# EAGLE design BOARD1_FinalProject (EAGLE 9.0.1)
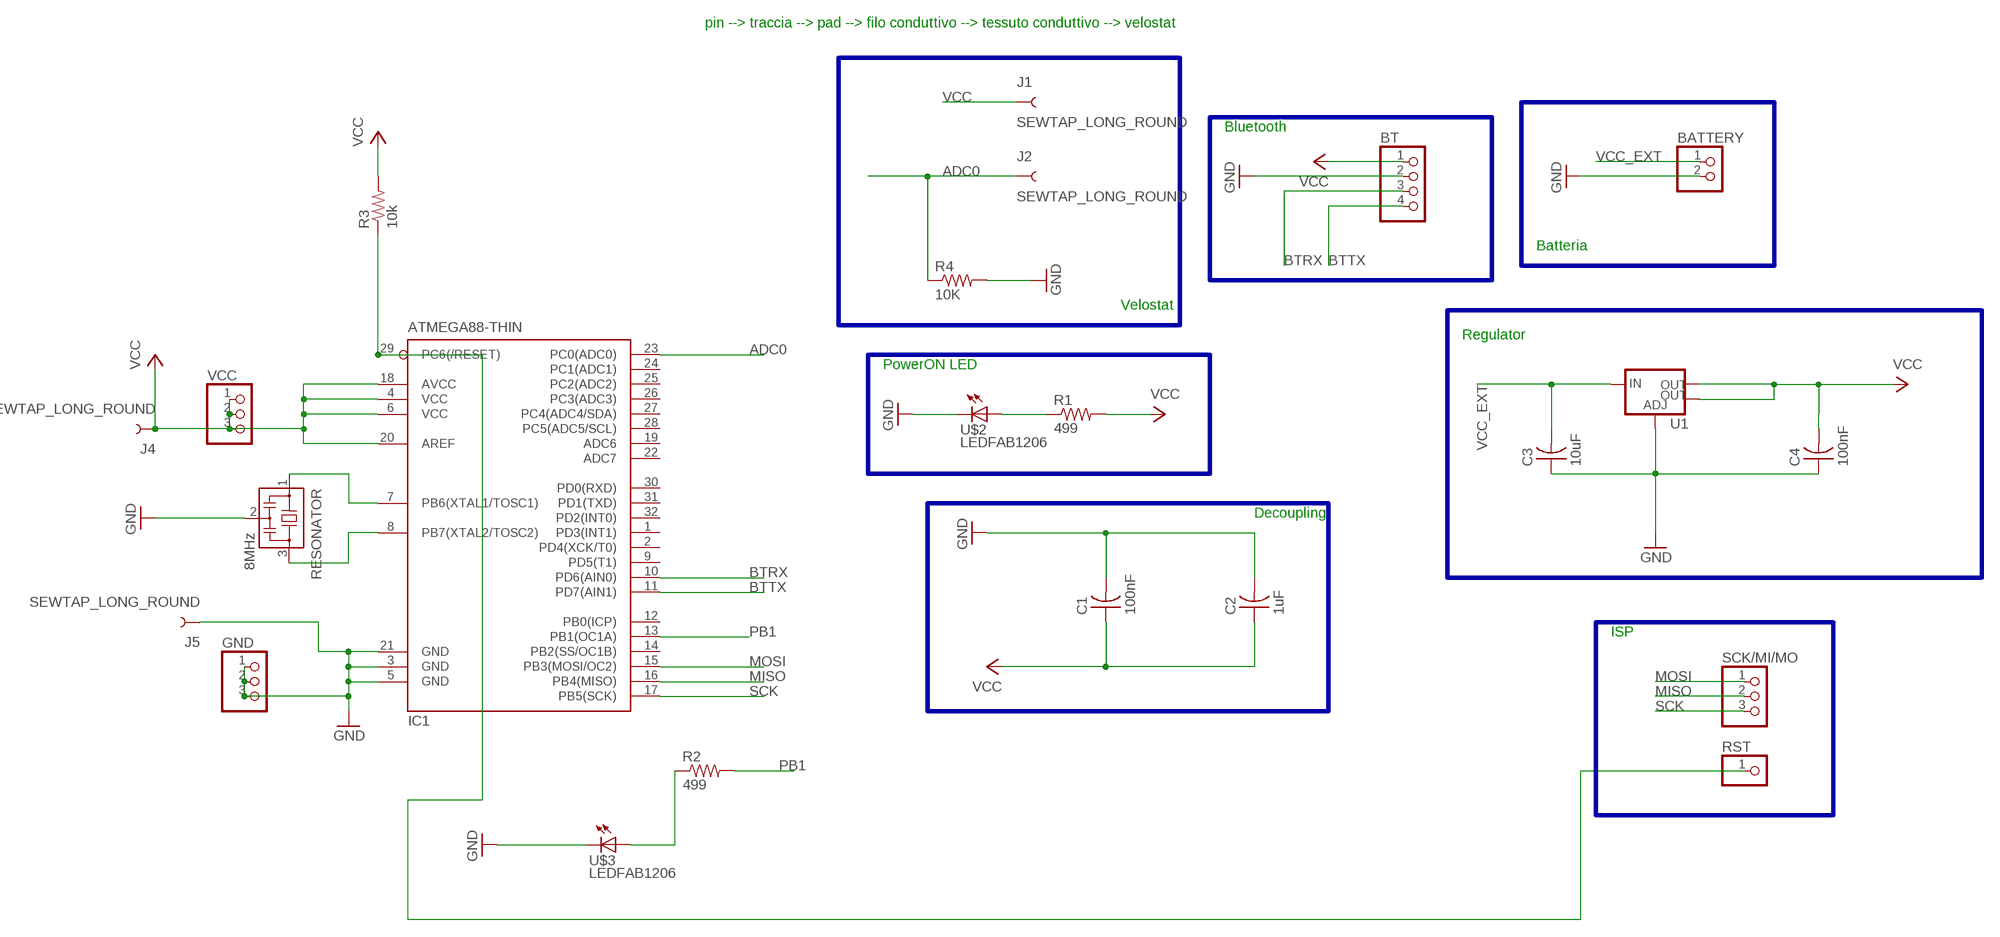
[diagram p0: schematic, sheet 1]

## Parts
BATTERY  PINHD-1X2  [1X02]
BT  PINHD-1X4  [1X04]
C1  100nF  CAP-US1206FAB  [C1206FAB]
C2  1uF  CAP-US1206FAB  [C1206FAB]
C3  10uF  CAP-US1206FAB  [C1206FAB]
C4  100nF  CAP-US1206FAB  [C1206FAB]
GND  PINHD-1X3  [1X03]
IC1  ATMEGA88-THIN  [TQFP32-08THIN]
J1  SEWTAP_LONG_ROUND  [PETAL-LONG-2]
J2  SEWTAP_LONG_ROUND  [PETAL-LONG-2]
J4  SEWTAP_LONG_ROUND  [PETAL-LONG-2]
J5  SEWTAP_LONG_ROUND  [PETAL-LONG-2]
R1  499  RES-US1206FAB  [R1206FAB]
R2  499  RES-US1206FAB  [R1206FAB]
R3  10k  RES-US1206FAB  [R1206FAB]
R4  10K  RES-US1206FAB  [R1206FAB]
RESONATOR  8MHz  RESONATOR  [EFOBM]
RST  PINHD-1X1  [1X01]
SCK/MI/MO  PINHD-1X3  [1X03]
U1  V_REG_LM1117SOT223  [SOT223]
U$2  LEDFAB1206  [LED1206FAB]
U$3  LEDFAB1206  [LED1206FAB]
VCC  PINHD-1X3  [1X03]

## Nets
ADC0: IC1.23(PC0(ADC0)) J2.1 R4.1
BTRX: BT.3 IC1.10(PD6(AIN0))
BTTX: BT.4 IC1.11(PD7(AIN1))
GND: BATTERY.2 BT.2 C1.2 C2.2 C3.1 C4.1 GND.1 GND.2 GND.3 IC1.3(GND) IC1.5(GND) IC1.21(GND) J5.1 R4.2 RESONATOR.2 U1.1(ADJ) U$2.2(C) U$3.2(C)
MISO: IC1.16(PB4(MISO)) SCK/MI/MO.2
MOSI: IC1.15(PB3(MOSI/OC2)) SCK/MI/MO.1
N$2: IC1.29(PC6(/RESET)) R3.1 RST.1
N$4: R2.1 U$3.1(A)
N$5: R1.1 U$2.1(A)
N$7: IC1.7(PB6(XTAL1/TOSC1)) RESONATOR.1
N$8: IC1.8(PB7(XTAL2/TOSC2)) RESONATOR.3
PB1: IC1.13(PB1(OC1A)) R2.2
SCK: IC1.17(PB5(SCK)) SCK/MI/MO.3
VCC: BT.1 C1.1 C2.1 C4.2 IC1.4(VCC) IC1.6(VCC) IC1.18(AVCC) IC1.20(AREF) J1.1 J4.1 R1.2 R3.2 U1.2(OUT) U1.4(OUT) VCC.1 VCC.2 VCC.3
VCC_EXT: BATTERY.1 C3.2 U1.3(IN)
Unconnected: IC1.1(PD3(INT1)) IC1.2(PD4(XCK/T0)) IC1.9(PD5(T1)) IC1.12(PB0(ICP)) IC1.14(PB2(SS/OC1B)) IC1.19(ADC6) IC1.22(ADC7) IC1.24(PC1(ADC1)) IC1.25(PC2(ADC2)) IC1.26(PC3(ADC3)) IC1.27(PC4(ADC4/SDA)) IC1.28(PC5(ADC5/SCL)) IC1.30(PD0(RXD)) IC1.31(PD1(TXD)) IC1.32(PD2(INT0))

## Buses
B$1
B$2
B$4
B$5
B$6
B$8
B$3

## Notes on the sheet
- pin --> traccia --> pad --> filo conduttivo --> tessuto conduttivo --> velostat
- Bluetooth
- Batteria
- Velostat
- Regulator
- PowerON LED
- Decoupling
- ISP

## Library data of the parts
BATTERY = pinhead:PINHD-1X2: PIN HEADER
BT = pinhead:PINHD-1X4: PIN HEADER
C1-C4 = fab:CAP-US
GND SCK/MI/MO VCC = pinhead:PINHD-1X3: PIN HEADER
IC1 = fab:ATMEGA88-THIN
J1 J2 J4 J5 = LilyPad-Wearables:SEWTAP: SparkFun LilyPad Sew Taps
R1-R4 = fab:RES-US: Resistor (US Symbol)
RESONATOR = fab:RESONATOR
RST = pinhead:PINHD-1X1: PIN HEADER
U1 = fab:V_REG_LM1117: Voltage Regulator LM1117 Standard adjustable voltage regulator but in SMD form. Spark Fun Electronics SKU : COM-00595; PROD_ID: VREG-08170
U$2 U$3 = fab:LED: LED

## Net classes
0 default: clearance 0.205 mm

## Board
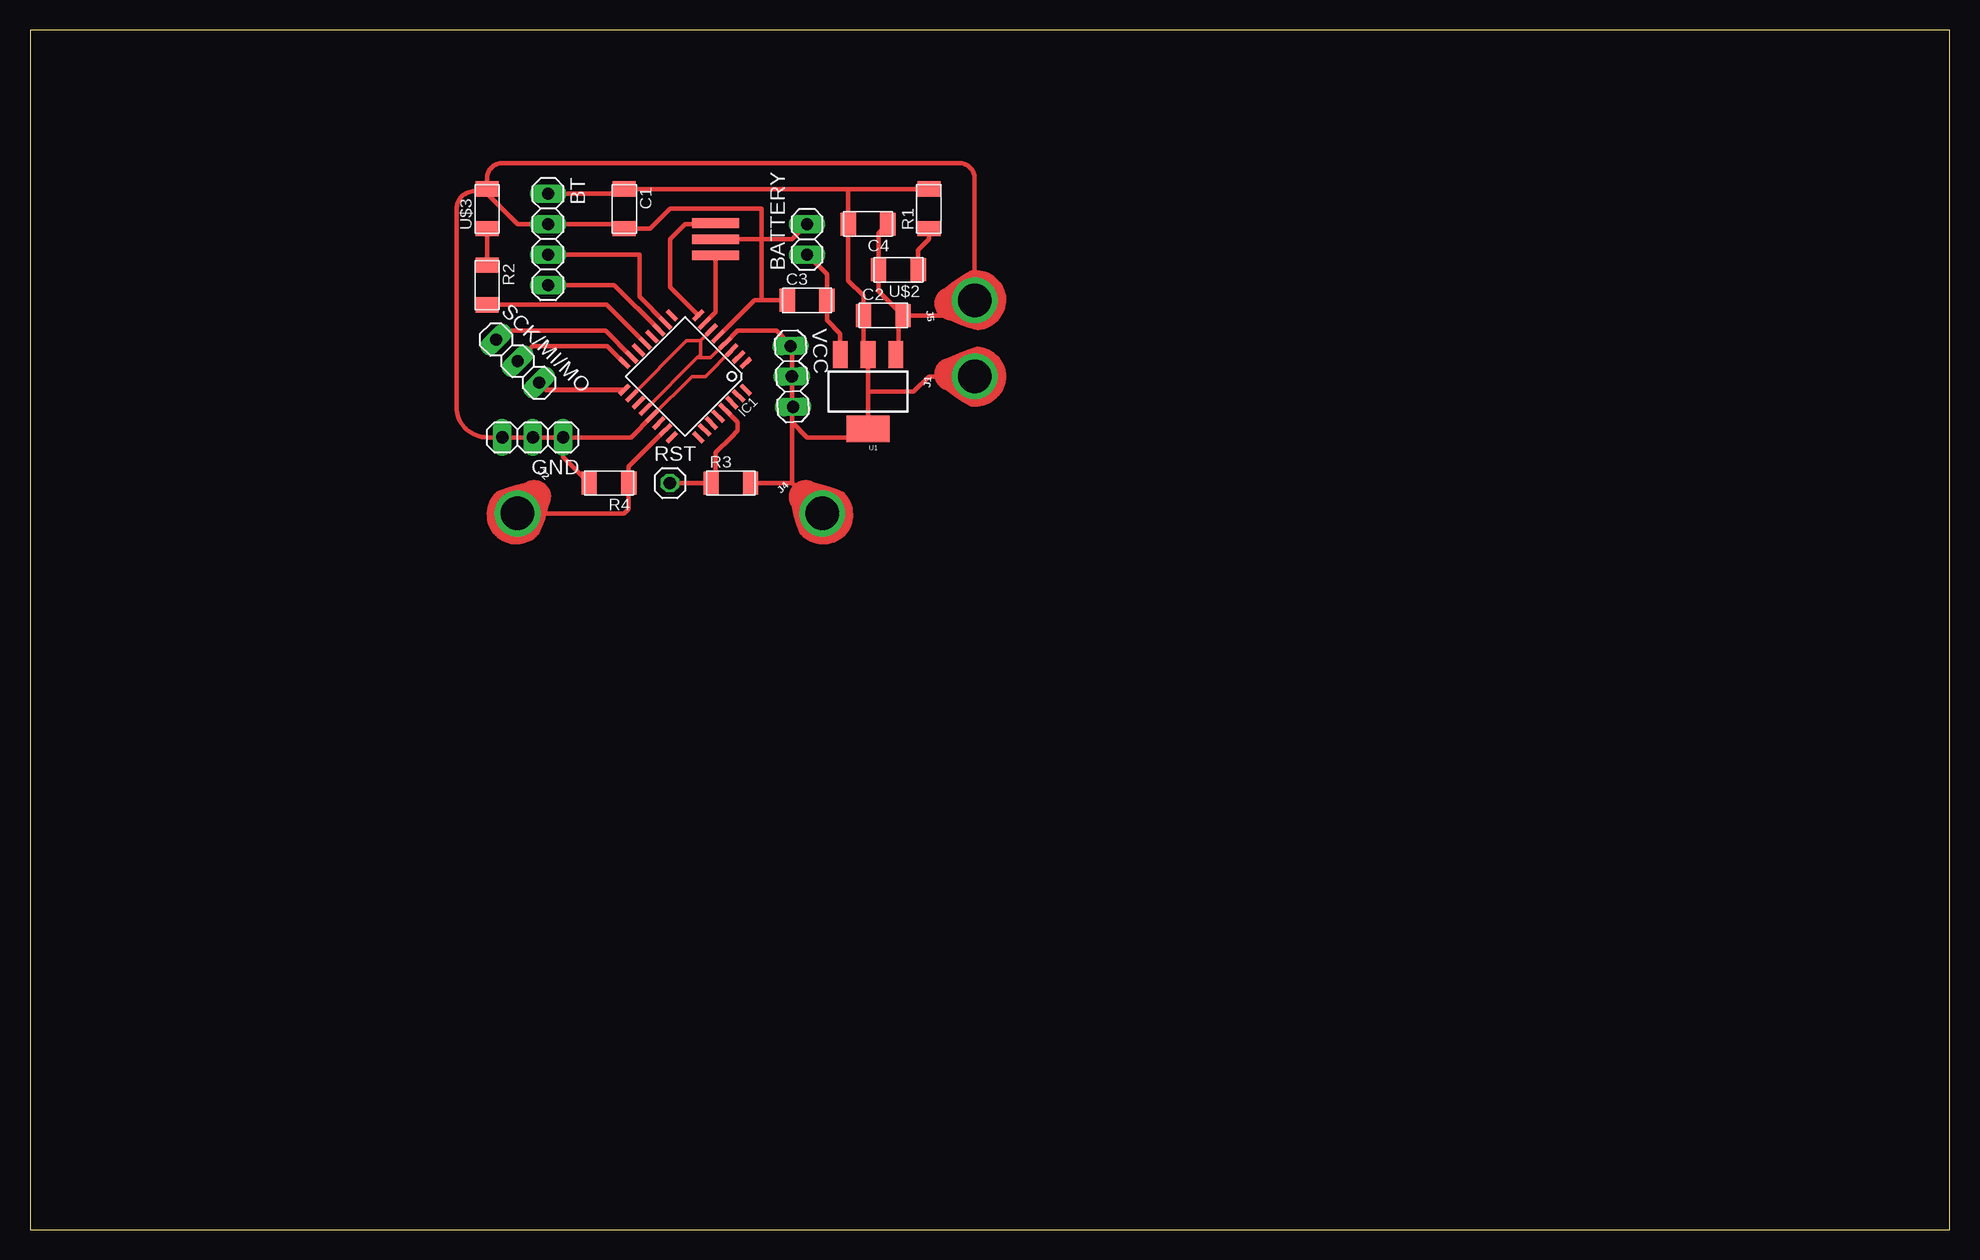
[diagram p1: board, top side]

Size 160 x 100 mm. Coordinates in mm from the lower left corner, seen from the top.
Outline: 0,0 160,0 160,100 0,100 0,0
Copper layers (1*16): Top 0.035mm / dielectric 1.5mm / Bottom 0.035mm
Design rules "default": minimum track width 6mil, minimum drill 0.35mm, track to track 6mil, track to pad 6mil, pad to pad 6mil, via to via 6mil, smd to smd 6mil, copper to edge 40mil, drill to drill 6mil, minimum pad ring 10mil, minimum via ring 8mil, stop-mask expansion 4mil, vias tented up to drill 0mil, thermal gap 10mil

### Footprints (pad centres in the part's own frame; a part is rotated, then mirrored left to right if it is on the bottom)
1X02 = drill 1.016 long: 1 -1.27,0; 2 1.27,0
1X04 = drill 1.016 long: 1 -3.81,0; 2 -1.27,0; 3 1.27,0; 4 3.81,0
C1206FAB = smd 1.27 x 1.905: 1 -1.651,0; 2 1.651,0
1X03 = drill 1.016 long: 1 -2.54,0; 2 0,0; 3 2.54,0
TQFP32-08THIN = smd 1.118 x 0.356: 1 -4.369,2.8; 8 -4.369,-2.8; 17 4.369,-2.8; 24 4.369,2.8 | smd 1.27 x 0.356: 2 -4.293,2; 3 -4.293,1.2; 4 -4.293,0.4; 5 -4.293,-0.4; 6 -4.293,-1.2; 7 -4.293,-2; 18 4.293,-2; 19 4.293,-1.2; 20 4.293,-0.4; 21 4.293,0.4; 22 4.293,1.2; 23 4.293,2 | smd 0.356 x 1.118: 9 -2.8,-4.369; 16 2.8,-4.369; 25 2.8,4.369; 32 -2.8,4.369 | smd 0.356 x 1.27: 10 -2,-4.293; 14 1.2,-4.293; 15 2,-4.293; 26 2,4.293; 27 1.2,4.293; 31 -2,4.293 | smd 0.35 x 1.27: 11 -1.2,-4.293; 12 -0.4,-4.293; 13 0.4,-4.293; 28 0.4,4.293; 29 -0.4,4.293; 30 -1.2,4.293
PETAL-LONG-2 = drill 2.794: 1 0,0
R1206FAB = smd 1.27 x 1.905: 1 -1.651,0; 2 1.651,0
EFOBM = smd 0.8 x 3.9: 1 -1.35,0; 2 0,0; 3 1.35,0
1X01 = drill 1.016 octagon: 1 0,0
SOT223 = smd 1.219 x 2.235: 1 -2.311,-3.099; 2 0,-3.099; 3 2.311,-3.099 | smd 3.6 x 2.2: 4 0,3.099
LED1206FAB = smd 1.27 x 1.905: 1 -1.651,0; 2 1.651,0

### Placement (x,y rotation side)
BATTERY  64.77,82.55 90 top
BT  43.18,82.55 270 top
C1  49.53,85.09 270 top
C2  71.12,76.2 0 top
C3  64.77,77.47 0 top
C4  69.85,83.82 180 top
GND  41.91,66.04 180 top
IC1  54.61,71.12 225 top
J1  78.74,71.12 84.8 top
J2  40.64,59.69 315 top
J4  66.04,59.69 45 top
J5  78.74,77.47 98 top
R1  74.93,85.09 90 top
R2  38.1,78.74 270 top
R3  58.42,62.23 0 top
R4  48.26,62.23 180 top
RESONATOR  57.15,82.55 90 top
RST  53.34,62.23 0 top
SCK/MI/MO  40.64,72.39 315 top
U1  69.85,69.85 180 top
U$2  72.39,80.01 180 top
U$3  38.1,85.09 90 top
VCC  63.5,71.12 272.4 top

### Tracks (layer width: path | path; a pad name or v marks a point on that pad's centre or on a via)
ADC0
  Top 0.356: IC1.23 49.91,63.59 R4.1 49.91,60.07 49.53,59.69 J2.1
BTRX
  Top 0.356: BT.3 50.8,81.28 50.8,77.76 IC1.10
BTTX
  Top 0.356: IC1.11 48.69,78.74 BT.4
GND
  Top 0.152: C2.2 72.39,76.2
  Top 0.305: IC1.21 55.18,71.12 56.31,71.12 IC1.3
  Top 0.356: IC1.21 50.1,66.04 GND.1 | 37.91,86.55 37.02,86.55 arc90 35.56,85.09 35.56,68.58 arc90 38.1,66.04 GND.3 GND.2 GND.1 | GND.1 44.45,64.39 R4.2 | 60.96,82.55 60.96,85.09 53.34,85.09 51.69,83.44 C1.2 49.53,83.82 | 60.96,82.55 RESONATOR.2 | 60.96,82.55 63.5,82.55 BATTERY.2 | C3.1 60.96,77.47 | 60.96,77.47 60.39,77.47 IC1.5 | 60.96,77.47 60.96,82.55 | U1.1 72.39,73.18 72.39,76.2 | C4.1 70.74,83.06 U$2.2 70.74,78.23 C2.2 77.47,76.2 J5.1 78.74,87.63 arc90 77.47,88.9 39.37,88.9 arc90 38.1,87.63 U$3.2 38.1,86.36 40.64,83.82 BT.2 49.15,83.82
  Top 0.406: U$3.2 37.91,86.55 37.72,86.36 | 49.15,83.82 C1.2
MISO
  Top 0.356: IC1.16 48.11,73.66 41.91,73.66 SCK/MI/MO.2
MOSI
  Top 0.356: SCK/MI/MO.1 39.59,74.93 47.97,74.93 IC1.15
N$2
  Top 0.356: RST.1 R3.1 | 57.15,62.61 57.15,64.77 58.42,66.04 58.99,66.61 58.99,67.31 IC1.29
  Top 0.406: R3.1 57.15,62.61
N$4
  Top 0.356: R2.1 U$3.1
  Top 0.406: 38.48,83.06 U$3.1
N$5
  Top 0.356: U$2.1 74.04,81.66 74.93,82.55 R1.1
N$7
  Top 0.356: IC1.7 57.15,76.49 RESONATOR.1
N$8
  Top 0.305: IC1.8 55.88,76.35
  Top 0.356: RESONATOR.3 57.07,83.82 54.61,83.82 53.34,82.55 53.34,78.57 IC1.8
PB1
  Top 0.356: 38.48,77.09 48.08,77.09 IC1.13
  Top 0.406: 38.48,77.09 R2.2
SCK
  Top 0.406: SCK/MI/MO.3 43.02,70.01 IC1.17
VCC
  Top 0.152: VCC.1 63.5,73.66
  Top 0.305: IC1.20 55.6,72.67 | 55.6,72.67 55.88,72.96 55.88,74.09 | 55.88,74.09 IC1.6 | IC1.18 54.75,74.09 55.88,74.09 | 55.6,72.67 56.73,72.67 IC1.4
  Top 0.356: BT.1 49.15,86.36 | C1.1 68.2,86.74 | 68.2,86.74 R1.2 | 68.2,86.74 C4.2 68.2,79.12 69.47,77.85 C2.1 69.47,73.33 | 69.85,67.31 U1.4 69.14,66.04 64.77,66.04 63.5,67.31 | 69.85,67.31 69.85,69.85 | 69.85,69.85 73.66,69.85 74.93,71.12 J1.1 | 69.85,69.85 U1.2 | IC1.4 58.99,74.93 62.23,74.93 63.5,73.66 VCC.2 63.5,68.48 | 68.58,66.04 69.85,67.31 | R3.2 63.5,62.23 | 63.5,62.23 J4.1 | 63.5,62.23 63.5,67.31 | VCC.3 63.5,68.48 | 63.5,68.48 63.5,67.31
  Top 0.406: 49.15,86.36 C1.1 49.91,86.36 | 69.85,66.04 U1.4 | 74.93,86.36 R1.2 | 69.85,76.2 C2.1 | U1.2 69.47,73.33
VCC_EXT
  Top 0.356: BATTERY.1 66.42,79.63 C3.2 66.42,75.82 67.54,74.7 U1.3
